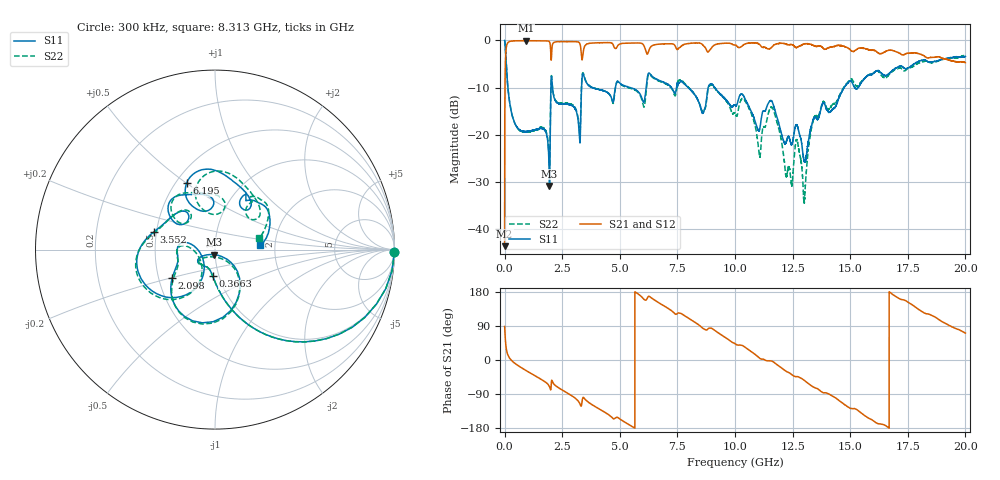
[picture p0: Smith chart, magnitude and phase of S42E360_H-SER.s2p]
!{S42E360}
!Johanson Technology Inc.
!www.johansontechnology.com
!Test Board Conditions:
!Substrate Type  RO4350B
!Substrate Thickness  50 mil
!Substrate Dk  3.66
!TL Type: GCPW
!TL Trace Width  60 mil
!TL Gap  10 mil
!Electrode orientation  Horizontal
!DUT TOPOLOGY	SERIES
!Mounting Pad LxW  14x55 mil
! Created Wed Nov 25 22:13:35 2020
# khz S ma R 50
! 2 Port Network Data from SP1.SP block
! freq  magS11  angS11  magS21  angS21  magS12  angS12  magS22  angS22
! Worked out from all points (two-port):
!   20001 points, 300 kHz to 20 GHz, reference 50 ohm
!   highest |S21| = -0.05 dB at 928.3 MHz (marker M1); lowest = -43.7 dB at 300 kHz (marker M2)
!   |S21| within 3 dB of the highest: 46.38 MHz to 2.007 GHz (1.961 GHz wide, 191 % of centre); 3.398 GHz to 17.26 GHz (13.87 GHz wide, 134 % of centre)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
!   lowest |S11| = -30.9 dB at 1.948 GHz (marker M3), VSWR 1.06, Z = 49.2 - j2.72 ohm
!   |S11| at or under -10 dB: 142.7 MHz to 2.01 GHz (1.868 GHz wide, 173 % of centre); 2.078 GHz to 3.339 GHz (1.262 GHz wide, 46.6 % of centre); 9.123 GHz to 14.74 GHz (5.616 GHz wide, 47.1 % of centre)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
!   |S22| runs from -34.5 to 0.0 dB; largest |S21 - S12| = 0.019
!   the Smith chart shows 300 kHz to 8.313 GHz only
!   S11 on the Smith chart (normalised r, x): 300 kHz: open; 366.3 MHz: 0.93, -0.28; 2.098 GHz: 0.59, -0.20; 3.552 GHz: 0.48, +0.11; 6.195 GHz: 0.57, +0.50; 8.313 GHz: 1.67, +0.08
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300  0.9998 -0.6  0.006546 88.5  0.006468 89.0  0.9997 -0.7
110300  0.3926 -70.8  0.9186 19.1  0.9186 19.1  0.3941 -70.9
366300  0.1487 -95.0  0.9872 -4.9  0.9886 -4.9  0.1483 -95.1
928300  0.1074 -117.0  0.9939 -27.7  0.9921 -27.7  0.1061 -118.9
1948300  0.02847 -104.0  0.967 -70.3  0.9666 -70.3  0.04105 -96.3
2098300  0.2856 -146.5  0.93 -60.1  0.9301 -60.1  0.2882 -144.1
3334300  0.2925 -121.8  0.6926 -120.5  0.6929 -120.5  0.3087 -122.4
3552300  0.3558 164.2  0.9107 -107.2  0.9114 -107.3  0.3601 166.7
4621300  0.2509 126.9  0.9438 -149.2  0.9434 -149.2  0.2497 123.8
6195300  0.4039 112.9  0.7158 163.4  0.7138 163.4  0.3803 104.7
6667300  0.38 69.8  0.9117 151.9  0.9101 151.8  0.3737 56.9
8313300  0.2521 5.2  0.9416 97.6  0.937 97.8  0.2528 14.6
1.00003e7  0.2053 -15.8  0.8949 43.1  0.8949 43.2  0.1685 -43.8
1.10593e7  0.1111 -25.2  0.9102 5.4  0.9116 5.4  0.05968 -67.9
1.16173e7  0.2227 -58.3  0.8588 -3.3  0.8613 -3.2  0.1934 -77.5
1.22133e7  0.08228 -52.4  0.916 -29.6  0.9198 -29.7  0.03664 -101.5
1.30063e7  0.05326 -38.5  0.9167 -53.5  0.9181 -53.8  0.01986 -39.9
1.33343e7  0.1277 -0.2  0.9009 -68.8  0.8999 -68.7  0.1214 -1.6
1.45373e7  0.2535 -17.7  0.8839 -108.2  0.8867 -107.7  0.2629 -30.5
1.66673e7  0.439 -98.2  0.7863 -178.5  0.7731 -178.8  0.4281 -95.0
1.80983e7  0.6171 -136.6  0.7056 128.3  0.7044 129.8  0.5885 -148.1
2e7  0.6769 167.1  0.5811 71.0  0.5803 72.1  0.6973 156.7
